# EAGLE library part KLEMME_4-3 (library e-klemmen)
Klemme 4 3
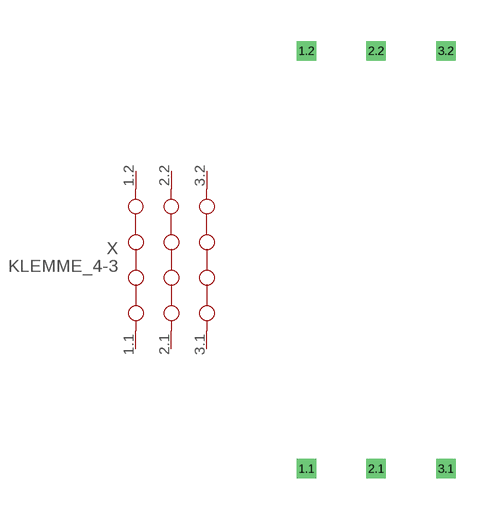
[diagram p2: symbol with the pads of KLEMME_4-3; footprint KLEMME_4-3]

Designator prefix X

## KLEMME_4-3  [KLEMME_4-3]
1.1  1.1  pas
1.2  1.2  pas
2.1  2.1  pas
2.2  2.2  pas
3.1  3.1  pas
3.2  3.2  pas

## Footprint KLEMME_4-3 (pad centres in mm)
Dummy
drill 0.2 pad 0.6 square: 1.1 -2.54,-7.62; 1.2 -2.54,7.62; 2.1 0,-7.62; 2.2 0,7.62; 3.1 2.54,-7.62; 3.2 2.54,7.62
